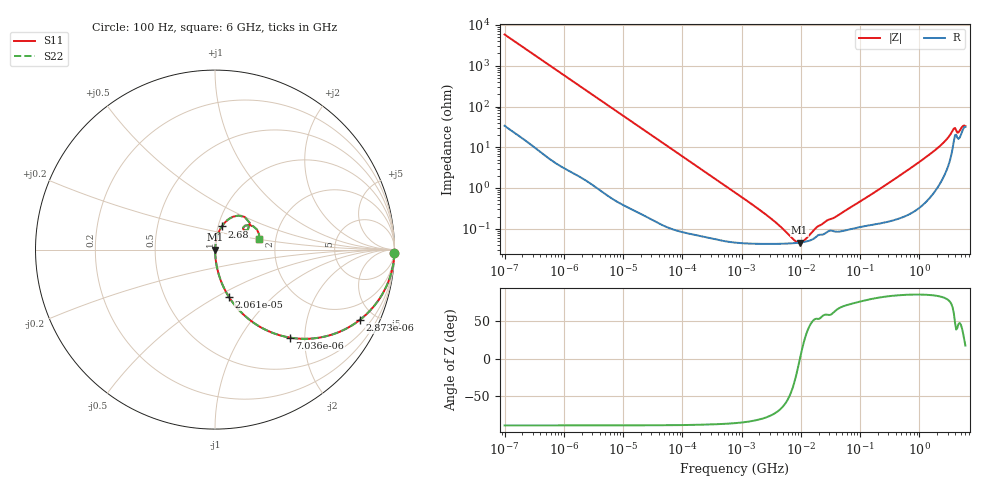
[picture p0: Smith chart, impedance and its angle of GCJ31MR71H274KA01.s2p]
!Murata Part Number: GCJ31MR71H274KA01
!These Parameters are Measured in Series Mode Connection
!Data Generated on Mar 13, 2026
!  o--ll--o
!Port1  Port2
!  o------o
!Operation Temp=25[degC], DC Bias Voltage=0[V]
!Freq. Start=100[Hz] Stop=6[GHz] 401[Steps]
# Hz S RI R 50
!Freq.(Hz) S11(Real) S11(Imag) S21(Real) S21(Imag) S12(Real) S12(Imag) S22(Real) S22(Imag)
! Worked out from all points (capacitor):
!   401 points, 100 Hz to 6 GHz, reference 50 ohm
!   read as one part in series: C = 271 nF near 109 Hz
!   lowest |Z| = 45.8 mohm at 9.506 MHz (marker M1)
!   series resonance near 9.674 MHz, so ESL is about 1 nH
!   S11 on the Smith chart (normalised r, x): 100 Hz: open; 2.873 kHz: 1.03, -4.13; 7.036 kHz: 1.01, -1.69; 20.61 kHz: 1.00, -0.58; 2.68 GHz: 1.04, +0.27; 6 GHz: 1.63, +0.20
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100  0.9996 -0.0171  0.000389 0.0171  0.000389 0.0171  0.9996 -0.0171
600  0.9893 -0.1006  0.0107 0.1006  0.0107 0.1006  0.9893 -0.1006
2008  0.8953 -0.3032  0.1047 0.3032  0.1047 0.3032  0.8953 -0.3032
2873  0.8082 -0.3907  0.1918 0.3907  0.1918 0.3907  0.8082 -0.3907
4702  0.6139 -0.4839  0.3861 0.4839  0.3861 0.4839  0.6139 -0.4839
7036  0.4171 -0.4901  0.5829 0.4901  0.5829 0.4901  0.4171 -0.4901
12041  0.1982 -0.3953  0.8018 0.3953  0.8018 0.3953  0.1982 -0.3953
20606  0.0792 -0.2661  0.9208 0.2661  0.9208 0.2661  0.0792 -0.2661
40335  0.0228 -0.1448  0.9772 0.1448  0.9772 0.1448  0.0228 -0.1448
129199  0.00291 -0.0463  0.9971 0.0463  0.9971 0.0463  0.00291 -0.0463
774597  0.000519 -0.00779  0.9995 0.00779  0.9995 0.00779  0.000519 -0.00779
2713602  0.000429 -0.00206  0.9996 0.00206  0.9996 0.00206  0.000429 -0.00206
7599586  0.000443 -0.000307  0.9996 0.000307  0.9996 0.000307  0.000443 -0.000307
9506416  0.000458 -2.18e-05  0.9995 2.18e-05  0.9995 2.18e-05  0.000458 -2.18e-05
1.137099e7  0.000476 0.000206  0.9995 -0.000206  0.9995 -0.000206  0.000476 0.000206
1.555665e7  0.000544 0.000632  0.9995 -0.000632  0.9995 -0.000632  0.000544 0.000632
2.662322e7  0.000798 0.00132  0.9992 -0.00132  0.9992 -0.00132  0.000798 0.00132
3.124326e8  0.0017 0.0135  0.9983 -0.0135  0.9983 -0.0135  0.0017 0.0135
2.679998e9  0.0381 0.1291  0.9619 -0.1291  0.9619 -0.1291  0.0381 0.1291
3.666503e9  0.1298 0.1896  0.8702 -0.1896  0.8702 -0.1896  0.1298 0.1896
4.586474e9  0.1558 0.1215  0.8442 -0.1215  0.8442 -0.1215  0.1558 0.1215
6e9  0.2444 0.0566  0.7556 -0.0566  0.7556 -0.0566  0.2444 0.0566
